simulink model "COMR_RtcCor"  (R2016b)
settings: Solver=FixedStepDiscrete  StartTime=0.0  StopTime=10.0  FixedStep=0.02  RelTol=1e-3  EnableMultiTasking=on

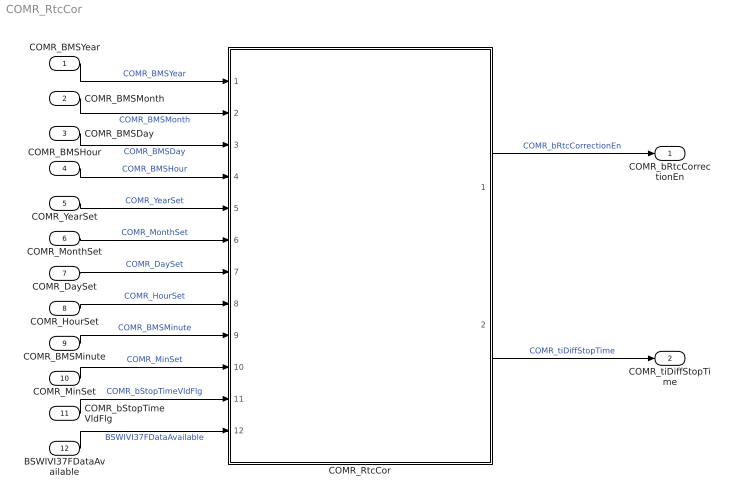
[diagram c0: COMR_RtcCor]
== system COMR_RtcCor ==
  COMR_BMSYear : Inport
  COMR_BMSMonth : Inport  Port=2
  COMR_BMSDay : Inport  Port=3
  COMR_BMSHour : Inport  Port=4
  COMR_YearSet : Inport  Port=5
  COMR_MonthSet : Inport  Port=6
  COMR_DaySet : Inport  Port=7
  COMR_HourSet : Inport  Port=8
  COMR_BMSMinute : Inport  Port=9
  COMR_MinSet : Inport  Port=10
  COMR_bStopTimeVldFlg : Inport  Port=11
  BSWIVI37FDataAvailable : Inport  Port=12
  COMR_RtcCor : Subsystem
  COMR_bRtcCorrectionEn : Outport
  COMR_tiDiffStopTime : Outport  Port=2
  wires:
  COMR_BMSYear/1 -> COMR_RtcCor/1(COMR_BMSYear)  "COMR_BMSYear"
  COMR_BMSMonth/1 -> COMR_RtcCor/2(COMR_BMSMonth)  "COMR_BMSMonth"
  COMR_BMSDay/1 -> COMR_RtcCor/3(COMR_BMSDay)  "COMR_BMSDay"
  COMR_BMSHour/1 -> COMR_RtcCor/4(COMR_BMSHour)  "COMR_BMSHour"
  COMR_YearSet/1 -> COMR_RtcCor/5(COMR_YearSet)  "COMR_YearSet"
  COMR_MonthSet/1 -> COMR_RtcCor/6(COMR_MonthSet)  "COMR_MonthSet"
  COMR_DaySet/1 -> COMR_RtcCor/7(COMR_DaySet)  "COMR_DaySet"
  COMR_HourSet/1 -> COMR_RtcCor/8(COMR_HourSet)  "COMR_HourSet"
  COMR_BMSMinute/1 -> COMR_RtcCor/9(COMR_BMSMinute)  "COMR_BMSMinute"
  COMR_MinSet/1 -> COMR_RtcCor/10(COMR_MinSet)  "COMR_MinSet"
  COMR_bStopTimeVldFlg/1 -> COMR_RtcCor/11(COMR_bStopTimeVldFlg)  "COMR_bStopTimeVldFlg"
  BSWIVI37FDataAvailable/1 -> COMR_RtcCor/12(BSWIVI37FDataAvailable)  "BSWIVI37FDataAvailable"
  COMR_RtcCor/1(COMR_bRtcCorrectionEn) -> COMR_bRtcCorrectionEn/1  "COMR_bRtcCorrectionEn"
  COMR_RtcCor/2(COMR_tiDiffStopTime) -> COMR_tiDiffStopTime/1  "COMR_tiDiffStopTime"

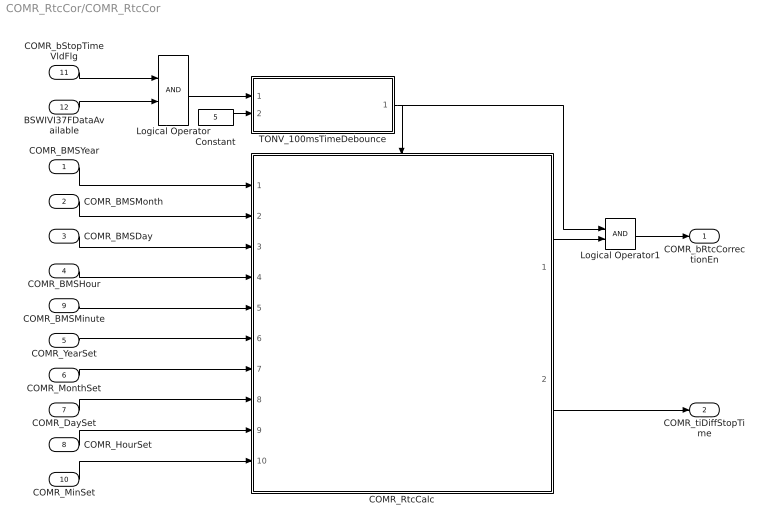
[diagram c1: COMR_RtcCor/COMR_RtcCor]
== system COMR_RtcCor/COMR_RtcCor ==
  COMR_BMSYear : Inport
  COMR_BMSMonth : Inport  Port=2
  COMR_BMSDay : Inport  Port=3
  COMR_BMSHour : Inport  Port=4
  COMR_YearSet : Inport  Port=5
  COMR_MonthSet : Inport  Port=6
  COMR_DaySet : Inport  Port=7
  COMR_HourSet : Inport  Port=8
  COMR_BMSMinute : Inport  Port=9
  COMR_MinSet : Inport  Port=10
  COMR_bStopTimeVldFlg : Inport  Port=11
  BSWIVI37FDataAvailable : Inport  Port=12
  COMR_RtcCalc : Subsystem
  Constant : Constant  Value=5
  Logical Operator : Logic  AllPortsSameDT=off  OutDataTypeStr=boolean
  Logical Operator1 : Logic  AllPortsSameDT=off  OutDataTypeStr=boolean
  TONV_100msTimeDebounce : Subsystem  TreatAsAtomicUnit=on  RTWFcnName=TONV_100msTimeDebounce  RTWFileName=SrvLib
  COMR_bRtcCorrectionEn : Outport
  COMR_tiDiffStopTime : Outport  Port=2
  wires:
  Logical Operator/1 -> TONV_100msTimeDebounce/1(u)
  COMR_bStopTimeVldFlg/1 -> Logical Operator/1
  BSWIVI37FDataAvailable/1 -> Logical Operator/2
  COMR_BMSYear/1 -> COMR_RtcCalc/1(COMR_BMSYear)
  COMR_BMSMonth/1 -> COMR_RtcCalc/2(COMR_BMSMonth)
  COMR_BMSDay/1 -> COMR_RtcCalc/3(COMR_BMSDay)
  COMR_BMSHour/1 -> COMR_RtcCalc/4(COMR_BMSHour)
  COMR_RtcCalc/1(COMR_bRtcCorrCond) -> Logical Operator1/2
  TONV_100msTimeDebounce/1(y) -> Logical Operator1/1, COMR_RtcCalc/Enable
  Constant/1 -> TONV_100msTimeDebounce/2(T)
  Logical Operator1/1 -> COMR_bRtcCorrectionEn/1
  COMR_RtcCalc/2(COMR_tiDiffStopTime) -> COMR_tiDiffStopTime/1
  COMR_BMSMinute/1 -> COMR_RtcCalc/5(COMR_BMSMinute)
  COMR_YearSet/1 -> COMR_RtcCalc/6(COMR_YearSet)
  COMR_MonthSet/1 -> COMR_RtcCalc/7(COMR_MonthSet)
  COMR_DaySet/1 -> COMR_RtcCalc/8(COMR_DaySet)
  COMR_HourSet/1 -> COMR_RtcCalc/9(COMR_HourSet)
  COMR_MinSet/1 -> COMR_RtcCalc/10(COMR_MinSet)

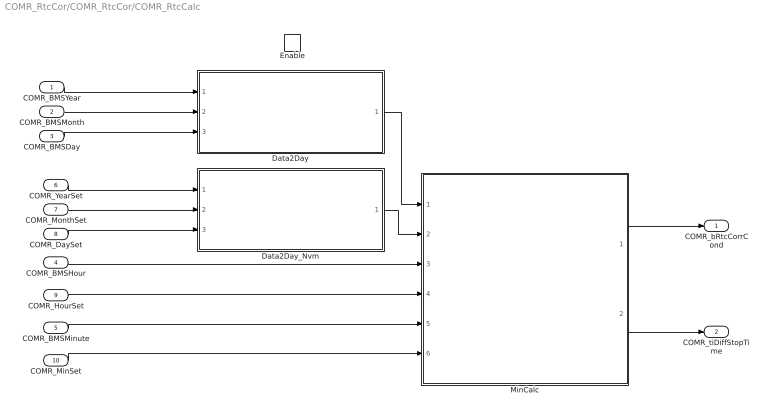
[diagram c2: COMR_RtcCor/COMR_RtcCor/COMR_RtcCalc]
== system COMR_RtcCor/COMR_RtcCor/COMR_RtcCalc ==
  COMR_BMSYear : Inport
  COMR_BMSMonth : Inport  Port=2
  COMR_BMSDay : Inport  Port=3
  COMR_BMSHour : Inport  Port=4
  COMR_BMSMinute : Inport  Port=5
  COMR_YearSet : Inport  Port=6
  COMR_MonthSet : Inport  Port=7
  COMR_DaySet : Inport  Port=8
  COMR_HourSet : Inport  Port=9
  COMR_MinSet : Inport  Port=10
  Enable : EnablePort
  Data2Day : Subsystem
  Data2Day_Nvm : Subsystem
  MinCalc : Subsystem
  COMR_bRtcCorrCond : Outport  InitialOutput=[0]
  COMR_tiDiffStopTime : Outport  Port=2
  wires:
  MinCalc/1(COMR_bRtcCorrCond) -> COMR_bRtcCorrCond/1
  COMR_BMSYear/1 -> Data2Day/1(BSER_tiYearSet)
  COMR_BMSDay/1 -> Data2Day/3(BSER_tiDaySet)
  COMR_BMSMonth/1 -> Data2Day/2(BSER_tiMonthSet)
  COMR_YearSet/1 -> Data2Day_Nvm/1(COMR_YearSet)
  COMR_MonthSet/1 -> Data2Day_Nvm/2(COMR_MonthSet)
  COMR_DaySet/1 -> Data2Day_Nvm/3(COMR_DaySet)
  COMR_BMSHour/1 -> MinCalc/3(COMR_BMSHour)
  COMR_HourSet/1 -> MinCalc/4(COMR_HourSet)
  COMR_MinSet/1 -> MinCalc/6(COMR_MinSet)
  COMR_BMSMinute/1 -> MinCalc/5(COMR_BMSMinute)
  Data2Day/1(BSER_tiDay) -> MinCalc/1(BSER_tiDay)
  Data2Day_Nvm/1(BSER_tiDaySet) -> MinCalc/2(BSER_tiDaySet)
  MinCalc/2(COMR_tiDiffStopTime) -> COMR_tiDiffStopTime/1

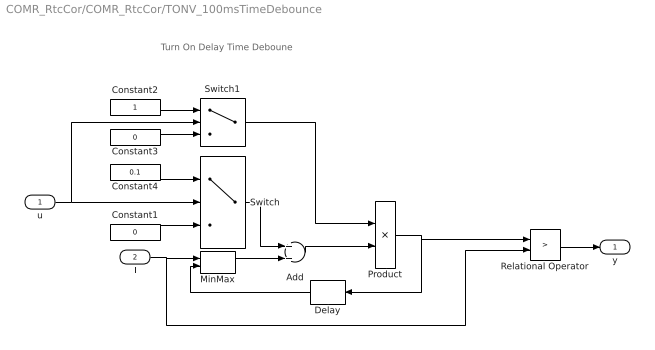
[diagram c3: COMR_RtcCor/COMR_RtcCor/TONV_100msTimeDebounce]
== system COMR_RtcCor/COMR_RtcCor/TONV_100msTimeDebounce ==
  note: Turn On Delay Time Deboune
  u : Inport
  T : Inport  Port=2
  Add : Sum
  Constant1 : Constant  Value=0  OutDataTypeStr=single
  Constant2 : Constant  OutDataTypeStr=uint8
  Constant3 : Constant  Value=0  OutDataTypeStr=uint8
  Constant4 : Constant  Value=0.1  OutDataTypeStr=single
  Delay : Delay  DelayLength=1  InitialCondition=0
  MinMax : MinMax  Inputs=2
  Product : Product  OutMin=[0]  OutMax=[65535]  OutDataTypeStr=single
  Relational Operator : RelationalOperator  Operator=>  OutDataTypeStr=boolean  RndMeth=Simplest
  Switch : Switch  Criteria=u2 ~= 0
  Switch1 : Switch  Criteria=u2 ~= 0
  y : Outport
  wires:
  Switch1/1 -> Product/1
  Constant3/1 -> Switch1/3
  Constant2/1 -> Switch1/1
  u/1 -> Switch1/2, Switch/2
  Constant4/1 -> Switch/1
  Constant1/1 -> Switch/3
  Add/1 -> Product/2
  Product/1 -> Relational Operator/1, Delay/1
  Switch/1 -> Add/1
  Delay/1 -> MinMax/2
  Relational Operator/1 -> y/1
  T/1 -> MinMax/1, Relational Operator/2
  MinMax/1 -> Add/2

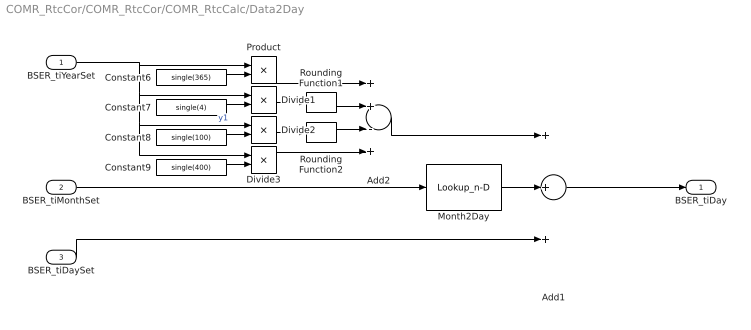
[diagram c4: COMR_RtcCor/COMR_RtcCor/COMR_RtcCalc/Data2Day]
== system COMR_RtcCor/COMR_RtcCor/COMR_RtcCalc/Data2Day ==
  BSER_tiYearSet : Inport
  BSER_tiMonthSet : Inport  Port=2
  BSER_tiDaySet : Inport  Port=3
  Add1 : Sum  Inputs=+++
  Add2 : Sum  Inputs=++-+
  Constant6 : Constant  Value=single(365)
  Constant7 : Constant  Value=single(4)
  Constant8 : Constant  Value=single(100)
  Constant9 : Constant  Value=single(400)
  Divide1 : Product  Inputs=*/
  Divide2 : Product  Inputs=*/
  Divide3 : Product  Inputs=*/
  Month2Day : Lookup_n-D  NumberOfTableDimensions=1  BreakpointsForDimension1=[1 2 3 4 5 6 7 8 9 10 11 12]  Table=[0 31 59 90 120 151 181 212 243 273 304 334]  InterpMethod=Flat  InternalRulePriority=Speed  OutDataTypeStr=single  RndMeth=Simplest
  Product : Product
  Rounding Function1 : Rounding
  Rounding Function2 : Rounding
  BSER_tiDay : Outport
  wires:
  Constant8/1 -> Divide2/2
  Divide2/1 -> Rounding Function2/1
  Add1/1 -> BSER_tiDay/1
  BSER_tiYearSet/1 -> Divide2/1, Divide3/1, Divide1/1, Product/1  "y1"
  BSER_tiMonthSet/1 -> Month2Day/1
  Constant6/1 -> Product/2
  Divide1/1 -> Rounding Function1/1
  Month2Day/1 -> Add1/2
  Constant7/1 -> Divide1/2
  Constant9/1 -> Divide3/2
  Product/1 -> Add2/1
  Rounding Function1/1 -> Add2/2
  Rounding Function2/1 -> Add2/3
  Divide3/1 -> Add2/4
  BSER_tiDaySet/1 -> Add1/3
  Add2/1 -> Add1/1

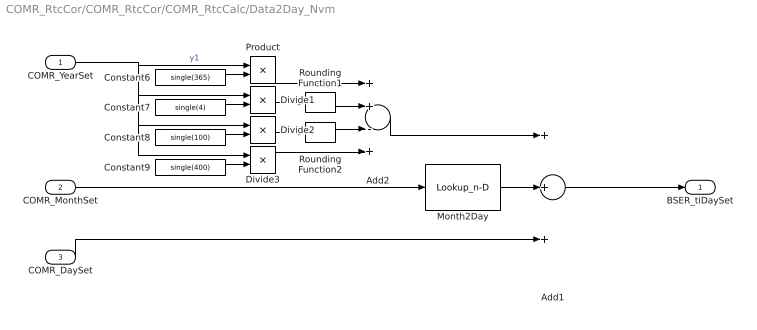
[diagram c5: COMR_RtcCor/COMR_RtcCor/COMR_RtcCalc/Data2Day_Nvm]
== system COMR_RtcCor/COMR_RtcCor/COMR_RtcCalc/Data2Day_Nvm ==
  COMR_YearSet : Inport
  COMR_MonthSet : Inport  Port=2
  COMR_DaySet : Inport  Port=3
  Add1 : Sum  Inputs=+++
  Add2 : Sum  Inputs=++-+
  Constant6 : Constant  Value=single(365)
  Constant7 : Constant  Value=single(4)
  Constant8 : Constant  Value=single(100)
  Constant9 : Constant  Value=single(400)
  Divide1 : Product  Inputs=*/
  Divide2 : Product  Inputs=*/
  Divide3 : Product  Inputs=*/
  Month2Day : Lookup_n-D  NumberOfTableDimensions=1  BreakpointsForDimension1=[1 2 3 4 5 6 7 8 9 10 11 12]  Table=[0 31 59 90 120 151 181 212 243 273 304 334]  InterpMethod=Flat  InternalRulePriority=Speed  OutDataTypeStr=single  RndMeth=Simplest
  Product : Product
  Rounding Function1 : Rounding
  Rounding Function2 : Rounding
  BSER_tiDaySet : Outport
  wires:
  Add2/1 -> Add1/1
  COMR_DaySet/1 -> Add1/3
  Divide3/1 -> Add2/4
  Rounding Function2/1 -> Add2/3
  Rounding Function1/1 -> Add2/2
  Product/1 -> Add2/1
  Constant9/1 -> Divide3/2
  Constant7/1 -> Divide1/2
  Month2Day/1 -> Add1/2
  Divide1/1 -> Rounding Function1/1
  Constant6/1 -> Product/2
  COMR_MonthSet/1 -> Month2Day/1
  COMR_YearSet/1 -> Product/1, Divide1/1, Divide3/1, Divide2/1  "y1"
  Add1/1 -> BSER_tiDaySet/1
  Divide2/1 -> Rounding Function2/1
  Constant8/1 -> Divide2/2

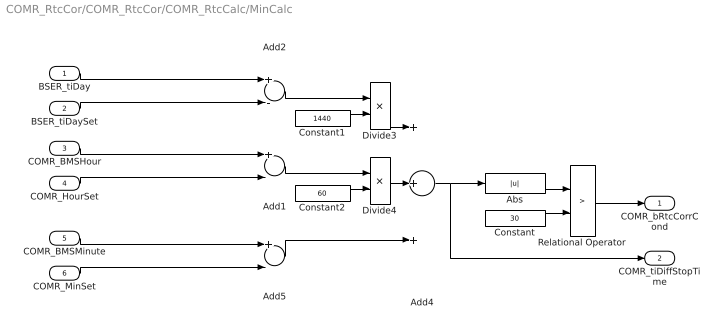
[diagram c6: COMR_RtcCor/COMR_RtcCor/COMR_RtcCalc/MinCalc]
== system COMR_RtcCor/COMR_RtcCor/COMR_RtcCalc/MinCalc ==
  BSER_tiDay : Inport
  BSER_tiDaySet : Inport  Port=2
  COMR_BMSHour : Inport  Port=3
  COMR_HourSet : Inport  Port=4
  COMR_BMSMinute : Inport  Port=5
  COMR_MinSet : Inport  Port=6
  Abs : Abs
  Add1 : Sum  Inputs=+-  OutDataTypeStr=int16
  Add2 : Sum  Inputs=+-  OutDataTypeStr=int16
  Add4 : Sum  Inputs=+++
  Add5 : Sum  Inputs=+-  OutDataTypeStr=int16
  Constant : Constant  Value=30
  Constant1 : Constant  Value=1440  OutDataTypeStr=uint16
  Constant2 : Constant  Value=60  OutDataTypeStr=uint16
  Divide3 : Product  Inputs=**  OutDataTypeStr=single
  Divide4 : Product  Inputs=**  OutDataTypeStr=single
  Relational Operator : RelationalOperator  Operator=>  OutDataTypeStr=boolean  RndMeth=Simplest
  COMR_bRtcCorrCond : Outport  InitialOutput=[0]
  COMR_tiDiffStopTime : Outport  Port=2
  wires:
  COMR_BMSHour/1 -> Add1/1
  COMR_HourSet/1 -> Add1/2
  Constant1/1 -> Divide3/2
  BSER_tiDay/1 -> Add2/1
  BSER_tiDaySet/1 -> Add2/2
  COMR_BMSMinute/1 -> Add5/1
  COMR_MinSet/1 -> Add5/2
  Add2/1 -> Divide3/1
  Constant2/1 -> Divide4/2
  Add1/1 -> Divide4/1
  Divide3/1 -> Add4/1
  Divide4/1 -> Add4/2
  Add5/1 -> Add4/3
  Constant/1 -> Relational Operator/2
  Abs/1 -> Relational Operator/1
  Add4/1 -> Abs/1, COMR_tiDiffStopTime/1
  Relational Operator/1 -> COMR_bRtcCorrCond/1
